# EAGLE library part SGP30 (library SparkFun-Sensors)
The SGP30 is a digital multi-pixel gas sensor designed for easy integration into air purifier, demand-controlled ventilation, and IoT applications.
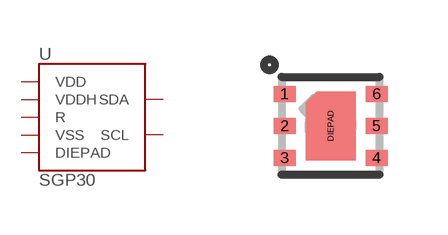
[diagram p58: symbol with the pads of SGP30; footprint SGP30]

Designator prefix U

## SGP30 (PROD_ID: IC-14776; VALUE: SGP30)  [SGP30]
1  VDD
2  VSS
3  SDA
4  R
5  VDDH
6  SCL
DIEPAD  DIEPAD

## Footprint SGP30 (pad centres in mm)
smd 0.55 x 0.4: 1 -1.15,0.8; 2 -1.15,0; 3 -1.15,-0.8; 4 1.15,-0.8; 5 1.15,0; 6 1.15,0.8
smd 0.305 x 0.61: DIEPAD 0,0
